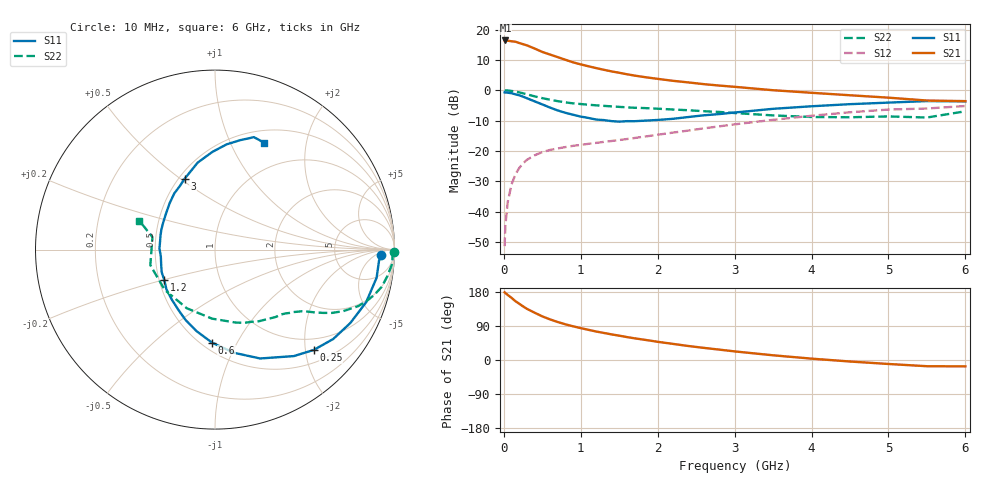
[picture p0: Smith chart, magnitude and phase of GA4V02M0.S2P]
! Infineon Technologies  Discrete & RF Semiconductors
! BF775
! Si NPN RF Bipolar Junction Transistor in SOT23
! VCE = 4 V  IC = 2 mA
! Common Emitter S-Parameters:  May  1996
# GHz  S  MA  R  50
!  f  S11  S21  S12  S22
! GHz  MAG  ANG  MAG  ANG  MAG  ANG  MAG  ANG
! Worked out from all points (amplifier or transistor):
!   36 points, 10 MHz to 6 GHz, reference 50 ohm
!   highest |S21| = 16.4 dB at 20 MHz (marker M1)
!   |S21| within 3 dB of that: start of sweep to 430.2 MHz
!   unconditionally stable (mu >= 1): 1.18 GHz to 3.655 GHz; 5.496679 GHz to 5.509128 GHz
!   at 250 MHz: K = 0.28, MSG = 19.6 dB, |S12| = -24.1 dB
!   at 1.4 GHz: K = 1.09, MAG = 9.6 dB, |S12| = -16.7 dB
!   at 6 GHz: K = 0.99, MSG = 0.8 dB, |S12| = -5.2 dB
!   S11 on the Smith chart (normalised r, x): 10 MHz: 21, -9; 250 MHz: 0.75, -2.17; 600 MHz: 0.56, -0.80; 1.2 GHz: 0.53, -0.20; 3 GHz: 0.54, +0.52; 6 GHz: 0.65, +1.35
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0.01  0.9232 -2.0  6.525 178.6  0.0027 86.8  0.9992 -0.8
0.02  0.9159 -3.9  6.612 176.5  0.0059 88.5  0.9893 -1.7
0.05  0.914 -9.9  6.557 171.8  0.0143 83.9  0.9908 -4.4
0.1  0.8918 -19.2  6.404 164.1  0.0281 78.9  0.9732 -8.5
0.15  0.8577 -28.5  6.307 155.3  0.0408 73.2  0.9517 -12.6
0.25  0.7842 -45.5  5.74 141.5  0.0626 64.8  0.8917 -18.8
0.3  0.7381 -53.5  5.488 135.0  0.0715 61.2  0.8571 -21.6
0.4  0.6566 -67.5  4.866 124.8  0.0848 55.7  0.7932 -25.6
0.5  0.5843 -79.6  4.279 115.1  0.0957 51.2  0.7415 -28.4
0.6  0.5188 -91.8  3.877 107.2  0.1039 48.6  0.6989 -30.3
0.7  0.4651 -102.9  3.513 100.3  0.1099 46.8  0.6613 -32.0
0.8  0.4252 -112.6  3.178 94.2  0.1158 45.6  0.6316 -33.3
0.9  0.3948 -120.7  2.883 88.9  0.1214 44.8  0.6085 -34.4
1.1  0.3497 -140.7  2.484 79.6  0.1311 44.6  0.5777 -36.8
1.2  0.3292 -149.2  2.318 75.2  0.1358 44.4  0.5641 -38.0
1.7  0.3093 171.7  1.744 57.2  0.1634 47.1  0.5142 -44.8
2.2  0.3386 143.8  1.43 42.5  0.2007 48.2  0.4815 -53.9
3  0.4296 113.2  1.139 22.7  0.2743 45.5  0.4215 -74.5
3.5  0.4945 101.2  1.001 12.4  0.3257 41.4  0.3851 -92.4
4.5  0.5899 83.7  0.827 -4.0  0.4341 29.4  0.359 -141.3
5.5  0.6629 70.9  0.677 -16.4  0.5004 13.3  0.3554 168.7
6  0.6557 65.3  0.662 -16.8  0.5501 8.8  0.4503 159.2
